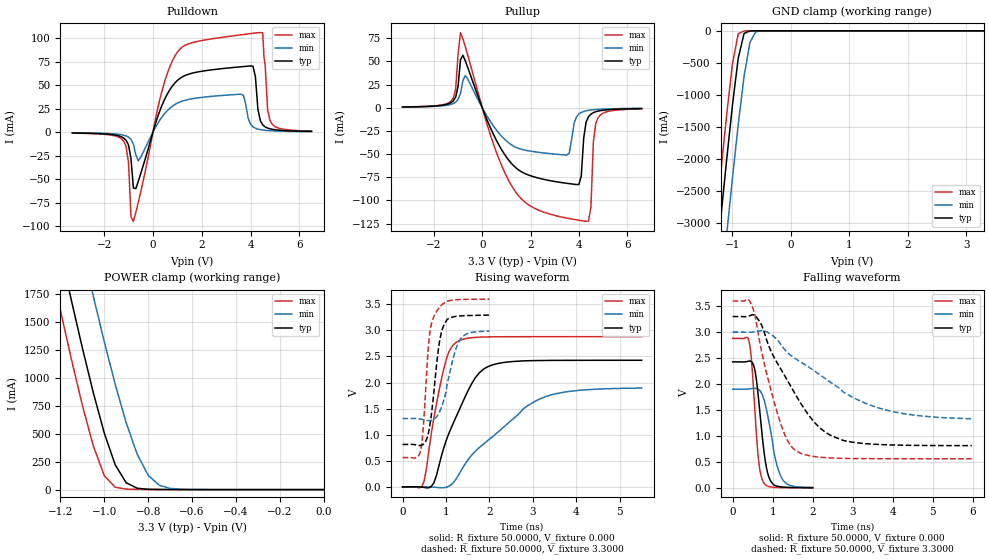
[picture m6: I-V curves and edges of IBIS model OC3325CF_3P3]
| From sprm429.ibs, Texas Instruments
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|   Model OC3325CF_3P3
[Model]   OC3325CF_3P3
Model_type   3-state
Polarity   Non-Inverting
Enable   Active-Low
Vmeas =   1.2500V
Cref =  15.0000pF
Rref = 100.0000M
Vref =  0.000V
C_comp   3.2113pF   3.3653pF   3.1996pF
[Temperature Range]   25.0000   0.1250k   -40.0000
[Pullup Reference]   3.3000V   3.0000V   3.6000V
[Pulldown Reference]   0.000V   0.000V   0.000V
[POWER Clamp Reference]   3.3000V   3.0000V   3.6000V
[GND Clamp Reference]   0.000V   0.000V   0.000V
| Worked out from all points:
|   slope of the pulldown table from 0 to 0.495 V, typ, clamps not added: 13.9 ohm
|   slope of the pullup table from 0 to 0.495 V, typ, clamps not added: 16.3 ohm
|   GND clamp passes 1 mA (typ) near -0.68 V on its own axis
|   POWER clamp passes 1 mA (typ) near -0.74 V on its own axis
|   rising waveform, R_fixture 50.0000, V_fixture 0.000: 20-80 % time 705ps typ, 1.41ns min, 376ps max; typ from 0 V to 2.43 V
|   rising waveform, R_fixture 50.0000, V_fixture 3.3000: 20-80 % time 203ps typ, 288ps min, 155ps max; typ from 0.814 V to 3.29 V
|   falling waveform, R_fixture 50.0000, V_fixture 0.000: 20-80 % time 207ps typ, 285ps min, 156ps max; typ from 2.43 V to 0.004 V
|   falling waveform, R_fixture 50.0000, V_fixture 3.3000: 20-80 % time 1.12ns typ, 1.92ns min, 597ps max; typ from 3.3 V to 0.814 V
[Pulldown]
| voltage   I(typ)   I(min)   I(max)
-3.3V     -858uA     -615uA     -1.004mA
-1.2V     -6.161mA   -3.225mA   -9.459mA
-800mV    -59.29mA   -12.78mA   -94.67mA
-600mV    -52.16mA   -30.52mA   -74.44mA
300mV     23.94mA    13.54mA    36.73mA
1V        54.91mA    30.86mA    84.97mA
3.6V      69.44mA    40.27mA    103.4mA
4.1V      70.14mA    5.645mA    105mA
4.4V      12.22mA    2.696mA    105.8mA
4.5V      7.744mA    2.284mA    105.4mA
4.8V      3.553mA    1.558mA    12.25mA
6.5V      840uA      548uA      1.177mA
|   6.6000   0.8040mA   0.5270mA   1.1170mA
[Pullup]
| voltage   I(typ)   I(min)   I(max)
-3.3V     804uA      687uA      859uA
-1.3V     5.391mA    3.609mA    6.959mA
-900mV    51.9mA     15.62mA    81.15mA
600mV     -35.88mA   -24.51mA   -49.07mA
1.7V      -70.21mA   -45.37mA   -100.4mA
3.5V      -81.59mA   -51.02mA   -119.1mA
4V        -82.91mA   -6.759mA   -121.4mA
4.3V      -15.54mA   -3.316mA   -122.6mA
4.5V      -6.854mA   -2.452mA   -107.1mA
4.6V      -5.293mA   -2.166mA   -37.37mA
4.8V      -3.612mA   -1.755mA   -10.57mA
6.6V      -915uA     -641uA     -1.25mA
[GND_clamp]
| voltage   I(typ)   I(min)   I(max)
-3.3V     -23.4A     -24.49A    -22.76A
-1.3V     -3.859A    -5.036A    -3.154A
-1.2V     -2.93A     -4.106A    -2.224A
-1.1V     -2.025A    -3.192A    -1.329A
-1V       -1.167A    -2.304A    -520.3mA
-900mV    -426.9mA   -1.461A    -45.96mA
-800mV    -40.65mA   -709.1mA   -2.555mA
-700mV    -1.225mA   -180.1mA   -233.9uA
-600mV    -46.8uA    -15.89mA   -13.11uA
-400mV    -100.8nA   -51.63uA   -11.56nA
3.3V      228.2pA    876.1nA    209.2pA
[POWER_clamp]
| voltage   I(typ)   I(min)   I(max)
-3.3V     22.53A     23.34A     22.08A
-1.25V    2.586A     3.492A     2.054A
-1.2V     2.135A     3.04A      1.604A
-1.15V    1.695A     2.594A     1.168A
-1.05V    867.5mA    1.733A     390.3mA
-1V       506.5mA    1.325A     124.9mA
-950mV    221.4mA    942.3mA    20.88mA
-900mV    61.07mA    598.5mA    4.539mA
-850mV    12.29mA    317.3mA    2.127mA
-800mV    3.014mA    129mA      1.191mA
-750mV    1.14mA     39.91mA    598.9uA
0V        228.2pA    1.731nA    267.3pA
[Ramp]
| variable   typ   min   max
dV/dt_r   1.4559/0.6980n   1.1360/1.4548n   1.7275/0.3719n
dV/dt_f   1.4909/1.1097n   0.9924/1.9217n   1.8228/0.5914n
R_load = 50.0000
[Rising Waveform]
R_fixture = 50.0000
V_fixture = 0.000
V_fixture_min = 0.000
V_fixture_max = 0.000
| time   V(typ)   V(min)   V(max)
0s        1.135nV    4.986nV    854.4pV
500ps     -10.82mV   1.305mV    121.2mV
722.2ps   81.61mV    -5.947mV   1.326V
944.4ps   737.1mV    -16.14mV   2.248V
1.111ns   1.116V     36.41mV    2.658V
1.278ns   1.427V     212.4mV    2.794V
1.611ns   2.007V     628.1mV    2.86V
1.889ns   2.27V      839.7mV    2.873V
3.111ns   2.421V     1.666V     2.879V
5.5ns     2.426V     1.893V     2.879V
[Rising Waveform]
R_fixture = 50.0000
V_fixture = 3.3000
V_fixture_min = 3.0000
V_fixture_max = 3.6000
| time   V(typ)   V(min)   V(max)
0s        813.5mV    1.309V     562mV
424.2ps   795.9mV    1.297V     732.4mV
484.8ps   821.6mV    1.286V     1.223V
606.1ps   1.074V     1.27V      2.792V
666.7ps   1.407V     1.276V     3.131V
767.7ps   2.216V     1.33V      3.341V
888.9ps   2.943V     1.513V     3.477V
1.03ns    3.211V     1.984V     3.558V
1.353ns   3.277V     2.853V     3.591V
2ns       3.292V     2.985V     3.598V
[Falling Waveform]
R_fixture = 50.0000
V_fixture = 0.000
V_fixture_min = 0.000
V_fixture_max = 0.000
| time   V(typ)   V(min)   V(max)
0s        2.427V     1.901V     2.879V
424.2ps   2.443V     1.908V     2.767V
484.8ps   2.421V     1.915V     2.327V
545.5ps   2.304V     1.918V     1.617V
646.5ps   1.722V     1.897V     548mV
767.7ps   801.4mV    1.744V     110.2mV
929.3ps   164.4mV    1.181V     22.54mV
1.071ns   42.67mV    550.5mV    9.517mV
1.232ns   18.62mV    183.3mV    6.171mV
2ns       3.7mV      8.131mV    1.359mV
[Falling Waveform]
R_fixture = 50.0000
V_fixture = 3.3000
V_fixture_min = 3.0000
V_fixture_max = 3.6000
| time   V(typ)   V(min)   V(max)
0s        3.3V       3V         3.6V
388.9ps   3.304V     2.997V     3.635V
500ps     3.336V     3V         3.475V
777.8ps   3.029V     3.027V     2.435V
1.167ns   2.338V     2.806V     1.319V
1.611ns   1.746V     2.468V     702.8mV
2.167ns   1.168V     2.187V     592.9mV
2.778ns   911.7mV    1.841V     568.2mV
4.056ns   826mV      1.462V     562.4mV
5.98ns    814.2mV    1.33V      562mV
